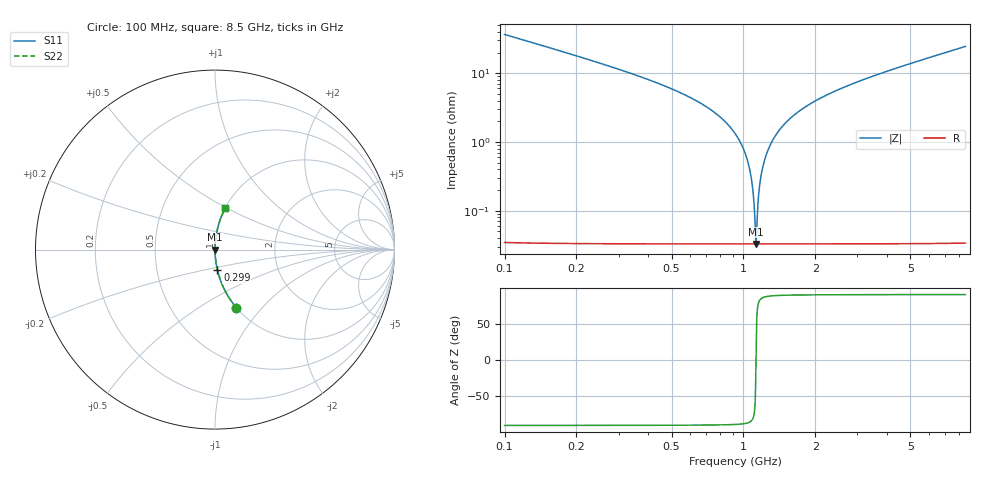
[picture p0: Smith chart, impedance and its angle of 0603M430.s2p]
! Created Wed Apr 18 16:51:37 2012
# hz S ma R 50
! 2 Port Network Data from SP1.SP block
! freq  magS11  angS11  magS21  angS21  magS12  angS12  magS22  angS22
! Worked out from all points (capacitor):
!   8401 points, 100 MHz to 8.5 GHz, reference 50 ohm
!   read as one part in series: C = 43.1 pF near 142 MHz
!   lowest |Z| = 32.9 mohm at 1.129 GHz (marker M1)
!   series resonance near 1.129 GHz, so ESL is about 460 pH
!   S11 on the Smith chart (normalised r, x): 100 MHz: 1.00, -0.73; 299 MHz: 1.00, -0.23; 8.5 GHz: 1.00, +0.49
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1e8  0.3439 -69.8  0.9387 20.1  0.9387 20.1  0.3439 -69.8
2.99e8  0.114 -83.3  0.9931 6.5  0.9931 6.5  0.114 -83.3
7.54e8  0.0271 -87.8  0.9993 1.6  0.9993 1.6  0.0271 -87.8
9.25e8  0.0131 -87.8  0.9996 0.8  0.9996 0.8  0.0131 -87.8
9.89e8  0.008668 -87.3  0.9996 0.5  0.9996 0.5  0.008668 -87.3
1.036e9  0.005615 -86.3  0.9997 0.3  0.9997 0.3  0.005615 -86.3
1.069e9  0.003564 -84.5  0.9997 0.2  0.9997 0.2  0.003564 -84.5
1.102e9  0.001592 -78.0  0.9997 0.1  0.9997 0.1  0.001592 -78.0
1.129e9  0.0003291 4.5  0.9997 -0.0  0.9997 -0.0  0.0003291 4.5
1.156e9  0.001606 78.1  0.9997 -0.1  0.9997 -0.1  0.001606 78.1
1.184e9  0.003157 83.9  0.9997 -0.2  0.9997 -0.2  0.003157 83.9
1.205e9  0.004304 85.4  0.9997 -0.2  0.9997 -0.2  0.004304 85.4
1.258e9  0.007127 87.0  0.9996 -0.4  0.9996 -0.4  0.007127 87.0
1.357e9  0.01214 87.8  0.9996 -0.7  0.9996 -0.7  0.01214 87.8
1.5e9  0.01887 87.9  0.9995 -1.1  0.9995 -1.1  0.01887 87.9
1.719e9  0.02835 87.7  0.9993 -1.6  0.9993 -1.6  0.02835 87.7
2.015e9  0.04008 87.2  0.9989 -2.3  0.9989 -2.3  0.04008 87.2
2.9e9  0.07125 85.7  0.9971 -4.1  0.9971 -4.1  0.07125 85.7
4.3e9  0.1156 83.2  0.993 -6.6  0.993 -6.6  0.1156 83.2
5.7e9  0.1576 80.8  0.9872 -9.1  0.9872 -9.1  0.1576 80.8
7.1e9  0.1984 78.5  0.9798 -11.4  0.9798 -11.4  0.1984 78.5
8.5e9  0.2382 76.1  0.9709 -13.8  0.9709 -13.8  0.2382 76.1
